ORGANIZATION_BLOCK OB 100
BEGIN

	// Check if OB-temp writing is enabled
	__FEATURE	1
	L		0
	<>D
	SPB isen

	// Enable OB-temp presets
	__FEATURE	1,	1
	// Reboot
	CALL		SFC -2 (
		REBOOT_TYPE := 1
	)

isen:	NOP		0

END_ORGANIZATION_BLOCK


ORGANIZATION_BLOCK OB 1
VAR_TEMP
	OB1_EV_CLASS		: BYTE
	OB1_SCAN_1		: BYTE
	OB1_PRIORITY		: BYTE
	OB1_OB_NUMBR		: BYTE
	OB1_RESERVED_1		: BYTE
	OB1_RESERVED_2		: BYTE
	OB1_PREV_CYCLE		: INT
	OB1_MIN_CYCLE		: INT
	OB1_MAX_CYCLE		: INT
	OB1_DATE_TIME		: DATE_AND_TIME
END_VAR
BEGIN

	L		#OB1_EV_CLASS
	__ASSERT==	__ACCU 1,	B#16#11

	L		#OB1_SCAN_1
	__ASSERT==	__ACCU 1,	B#16#03

	L		#OB1_PRIORITY
	__ASSERT==	__ACCU 1,	B#16#01

	L		#OB1_OB_NUMBR
	__ASSERT==	__ACCU 1,	B#16#01

	L		#OB1_RESERVED_1
	__ASSERT==	__ACCU 1,	B#16#00

	L		#OB1_RESERVED_2
	__ASSERT==	__ACCU 1,	B#16#00

	L		#OB1_PREV_CYCLE
	__ASSERT<=	__ACCU 1,	W#16#7FFF

	L		#OB1_MIN_CYCLE
	__ASSERT<=	__ACCU 1,	W#16#7FFF

	L		#OB1_MAX_CYCLE
	__ASSERT<=	__ACCU 1,	W#16#7FFF

	LAR1		P##OB1_DATE_TIME
	L		B [AR1, P#0.0]	// year
	T		MB 0
	CALL		FC 1 (BCD_BYTE := MB 0)
	__ASSERT>=	MB 0,		B#16#13
	L		B [AR1, P#1.0]	// month
	T		MB 0
	CALL		FC 1 (BCD_BYTE := MB 0)
	__ASSERT<=	MB 0,		B#16#12
	L		B [AR1, P#2.0]	// day
	T		MB 0
	CALL		FC 1 (BCD_BYTE := MB 0)
	__ASSERT<=	MB 0,		B#16#31
	L		B [AR1, P#3.0]	// hour
	T		MB 0
	CALL		FC 1 (BCD_BYTE := MB 0)
	__ASSERT<=	MB 0,		B#16#24
	L		B [AR1, P#4.0]	// minute
	T		MB 0
	CALL		FC 1 (BCD_BYTE := MB 0)
	__ASSERT<=	MB 0,		B#16#60
	L		B [AR1, P#5.0]	// second
	T		MB 0
	CALL		FC 1 (BCD_BYTE := MB 0)
	__ASSERT<=	MB 0,		B#16#60
	L		B [AR1, P#6.0]	// millisecond upper
	T		MB 0
	CALL		FC 1 (BCD_BYTE := MB 0)
	L		B [AR1, P#7.0]	// millisecond lower / weekday
	T		MB 0
	CALL		FC 1 (BCD_BYTE := MB 0)
	L		MB 0
	UD		DW#16#0000000F
	__ASSERT>=	__ACCU 1,	1
	__ASSERT<=	__ACCU 1,	7

	__ASSERT<=	#OB1_PREV_CYCLE,	#OB1_MAX_CYCLE
	__ASSERT>=	#OB1_PREV_CYCLE,	#OB1_MIN_CYCLE
	__ASSERT>=	#OB1_MAX_CYCLE,		#OB1_MIN_CYCLE

END_ORGANIZATION_BLOCK


FUNCTION FC 1 : VOID
TITLE = Check whether BCD_BYTE is a valid BCD value
VAR_INPUT
	BCD_BYTE	: BYTE
END_VAR
BEGIN
	L		#BCD_BYTE
	UD		DW#16#0000000F
	__ASSERT<=	__ACCU 1,	9
	L		#BCD_BYTE
	SRD		4
	UD		DW#16#0000000F
	__ASSERT<=	__ACCU 1,	9
END_FUNCTION
